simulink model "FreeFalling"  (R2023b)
settings: Solver=VariableStepAuto  StartTime=0.0  StopTime=10.0  RelTol=1e-3

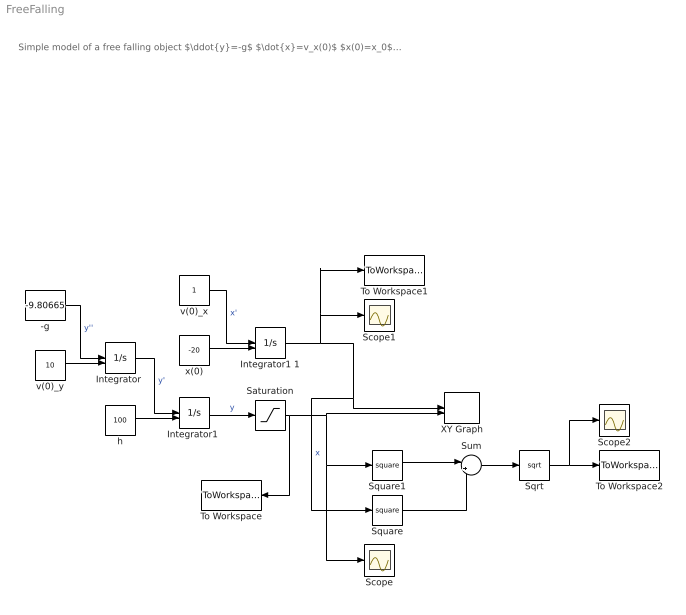
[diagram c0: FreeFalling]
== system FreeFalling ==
  note: Simple model of a free falling object $\ddot{y}=-g$ $\dot{x}=v_x(0)$ $x(0)=x_0$ $y(0)=h$ $\dot{y}(0)=v_{y}(0)$
  -g : Constant  Value=-9.80665
  "Integrator " : Integrator  InitialConditionSource=external
  "Integrator1 " : Integrator  InitialConditionSource=external
  Integrator1 1 : Integrator  InitialConditionSource=external
  Saturation : Saturate  UpperLimit=Inf  LowerLimit=0
  Scope : Scope
  Scope1 : Scope
  Scope2 : Scope
  Sqrt : Sqrt
  Square : Math  Operator=square
  Square1 : Math  Operator=square
  Sum : Sum  Inputs=|++
  To Workspace : ToWorkspace  VariableName=y  SaveFormat=Timeseries  SampleTime=-1
  To Workspace1 : ToWorkspace  VariableName=x  SaveFormat=Timeseries  SampleTime=-1
  To Workspace2 : ToWorkspace  VariableName=distance  SaveFormat=Timeseries  SampleTime=-1
  XY Graph : Record  FileSettingsInternal="{\"entries\":[{\"content\":{\"excelSettings\":{\"content\":{},\"type\":\"Streamout.ExcelSettings\"}},\"type\":\"Streamout.FileSettingStorage\",\"uuid\":\"\"}],\"packageUris\":[\"http:\\/\\/schema.mathworks.com\\/mf0\\/streamout_blocks\\/R2020a\"],\"version\":\"1.0\"}"  Layout=[1 1]  SignalsInternal="{\"entries\":[{\"content\":{\"signals\":[{\"content\":{\"blockPath\":[],\"dimensions\":[1],\"domain\":\"\",\"lineColor\":\"#a2142f\",\"plots\":[ 1 ],\"port\":1,\"sid\":[\"\"],\"signalID\":1,\"signalName\":\"x\"},\"type\":\"RecordBlkView.Signal\",\"uuid\":\"\"},{\"content\":{\"blockPath\":[],\"dimensions\":[1],\"domain\":\"\",\"lineColor\":\"#139fff\",\"plots\":[ 1 ],\"port\":2,\"sid\":[\"\"],\"signalID\":2,\"signalName\":\"Saturation\"},\"type\":\"RecordBlkView.Signal\"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"  VisualizationBindings="{\"xyplotplugin\":{\"info\":[{\"series\":[{\"bindingParametersList\":[{\"parameter\":\"X-Axis\",\"signalID\":1,\"signalName\":\"x\"},{\"parameter\":\"Y-Axis\",\"signalID\":2,\"signalName\":\"Saturation\"}],\"seriesID\":0}],\"subplotID\":1}]}}"  CompatibilityTag=XY
  h : Constant  Value=100
  v(0)_x : Constant
  v(0)_y : Constant  Value=10
  x(0) : Constant  Value=-20
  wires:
  -g/1 -> "Integrator "/1  "y''"
  "Integrator "/1 -> "Integrator1 "/1  "y'"
  v(0)_y/1 -> "Integrator "/2
  v(0)_x/1 -> Integrator1 1/1  "x'"
  h/1 -> "Integrator1 "/2
  x(0)/1 -> Integrator1 1/2
  "Integrator1 "/1 -> Saturation/1  "y"
  Integrator1 1/1 -> XY Graph/1, Square/1, Scope1/1, To Workspace1/1  "x"
  Saturation/1 -> XY Graph/2, Scope/1, Square1/1, To Workspace/1
  Square1/1 -> Sum/1
  Square/1 -> Sum/2
  Sum/1 -> Sqrt/1
  Sqrt/1 -> To Workspace2/1, Scope2/1
